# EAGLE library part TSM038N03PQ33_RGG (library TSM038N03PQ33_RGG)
MOSFET Power MOSFET, N-CHAN 30V, 80A, 3.8mOhm Source: Datasheet
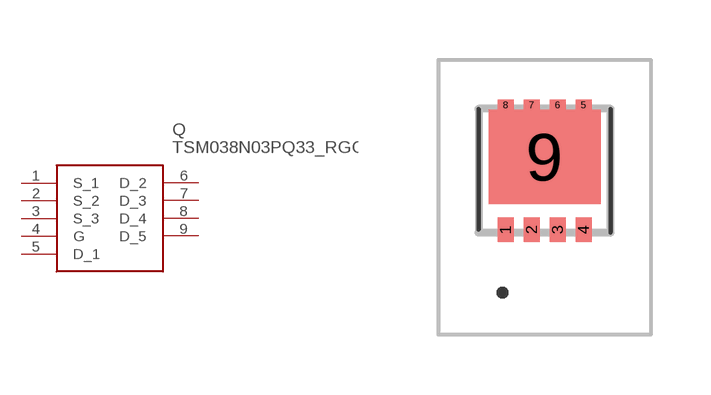
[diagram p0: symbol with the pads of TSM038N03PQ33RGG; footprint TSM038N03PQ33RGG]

Designator prefix Q

## TSM038N03PQ33_RGG (Arrow_Part_Number: TSM038N03PQ33 RGG; Arrow_Price-Stock: https://www.arrow.com/en/products/tsm038n03pq33rgg/taiwan-semiconductor; Description: MOSFET Power MOSFET, N-CHAN 30V, 80A, 3.8mOhm; Height: 0.8mm; Manufacturer_Name: Taiwan Semiconductor; Manufacturer_Part_Number: TSM038N03PQ33 RGG; Mouser_Part_Number: 821-TSM038N03PQ33RGG; Mouser_Price-Stock: https://www.mouser.co.uk/ProductDetail/Taiwan-Semiconductor/TSM038N03PQ33-RGG?qs=QEzMiVqgwc0dH14meb3EeQ%3D%3D)  [TSM038N03PQ33RGG]
1  S_1
2  S_2
3  S_3
4  G
5  D_1
6  D_2
7  D_3
8  D_4
9  D_5

## Footprint TSM038N03PQ33RGG (pad centres in mm)
TSM038N03PQ33 RGG-2
smd 0.4 x 0.6: 1 -0.975,-1.525; 2 -0.325,-1.525; 3 0.325,-1.525; 4 0.975,-1.525
smd 0.4 x 0.25: 5 0.975,1.6; 6 0.325,1.6; 7 -0.325,1.6; 8 -0.975,1.6
smd 2.8 x 2.35: 9 0,0.3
